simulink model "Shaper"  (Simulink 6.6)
settings: Solver=FixedStepDiscrete  StartTime=0.0  StopTime=1  FixedStep=0.001  RelTol=1e-3
PreLoadFcn:
  | load parameters
undefined symbols (not defined in the file or in its folder): f32_Traction_SlipShaperC, f32_Traction_SlipShaperDis, u32_Traction_SlipShaperOpt, u32_Traction_SlipShaperT

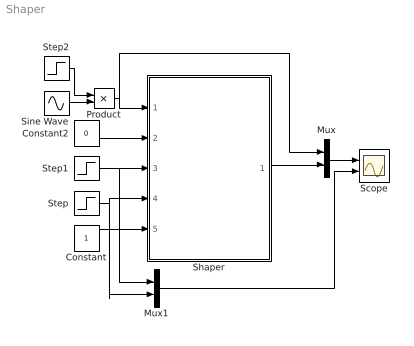
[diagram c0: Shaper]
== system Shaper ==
  Constant : Constant
  Constant2 : Constant  Value=0
  Mux : Mux  Inputs=2
  Mux1 : Mux  Inputs=2
  Product : Product
  Scope : Scope  NumInputPorts=2
  Shaper : Stateflow chart  TreatAsAtomicUnit=on
  Sine Wave : Sin  Amplitude=0.3  Bias=10  Frequency=2*pi  SampleTime=0
  Step : Step  Time=0.6  SampleTime=0
  Step1 : Step  Time=0.5  SampleTime=0
  Step2 : Step  Time=0.1  SampleTime=0
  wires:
  Constant/1 -> Shaper/5(EnableIn)
  Step/1 -> Shaper/4(Trigger), Mux1/2
  Constant2/1 -> Shaper/2(slip)
  Mux/1 -> Scope/1
  Shaper/1(out) -> Mux/2
  Step1/1 -> Shaper/3(CtrlActive), Mux1/1
  Mux1/1 -> Scope/2
  Product/1 -> Shaper/1(in), Mux/1
  Sine Wave/1 -> Product/2
  Step2/1 -> Product/1

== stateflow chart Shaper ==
  state Shaper [parallel]
    state PROCESS(N) [function]
      (junction 31) -> (junction 17)
      (junction 17) -> (junction 18) : [cnt < N] {j = MOD(j+u32_Traction_SlipShaperT[cnt],512); ... buf1[j] += f32_Traction_SlipShaperC[cnt+1]*(in-lev);}
      (junction 18) -> (junction 17) : {cnt++;}
      (junction 17) -> (junction 19)
      (default) -> (junction 31) : {cnt = 0;}
      (junction 30) -> (junction 19)
      (junction 20) -> (junction 30) : {cnt++;}
      (junction 30) -> (junction 20) : [cnt < N] {j = MOD(j+u32_Traction_SlipShaperT[cnt],512); ... buf2[j] += f32_Traction_SlipShaperC[cnt+1]*(in-lev);}
      (junction 31) -> (junction 30) : [bufSel]
    state c = MOD(a,b) [function]
      (default) -> (junction 33)
      (junction 33) -> (junction 34) : [a<b] {c=a;}
      (junction 33) -> (junction 34) : {c=a-b*floor(a/b);}
    state SHAPING /
      j = i;
      SETOUT();
      PROCESS(15);
      i = MOD(i+1,512);
      CtrlActiveOld = CtrlActive;
      EnableInOld = EnableIn;
    state SETOUT [function]
      (junction 21) -> (junction 22) : [bufSel] {tmp = f32_Traction_SlipShaperC[0] * (in-lev) + buf2[j] + lev; buf2[j] = 0;}
      (junction 21) -> (junction 22) : {tmp = f32_Traction_SlipShaperC[0] * (in-lev) + buf1[j] + lev; buf1[j] = 0;}
      (default) -> (junction 21)
      (junction 22) -> (junction 36) : {out = tmp;}
      (junction 22) -> (junction 36) : [u32_Traction_SlipShaperOpt && ... (tmp >= in - f32_Traction_SlipShaperDis)] {DisableShp = 1; out = in;}
    state b = SEL(a) [function]
      (default) -> (junction 28)
      (junction 28) -> (junction 29) : {b = 1; Pad1 = 1;}
      (junction 28) -> (junction 29) : [a] {b = 0; Pad2 = 1;}
    state DISABLED /
      out = in;
      CtrlActiveOld = CtrlActive;
      EnableInOld = EnableIn;
    (junction 15) -> (junction 37)
    (junction 16) -> (junction 15) : [(CtrlActive > CtrlActiveOld) ...  && bufAvailable] {ReadyToTrigg = 1;}
    (junction 15) -> SHAPING  : [ReadyToTrigg && Trigger] {lev = slip; bufSel = SEL(bufSel); ... bufAvailable--; ReadyToTrigg = 0; ... DisableShp = 0;}
    SHAPING  -> (junction 35)
    (junction 16) -> (junction 15) : [!CtrlActive] {ReadyToTrigg = 0;}
    (default) -> SHAPING 
    (junction 16) -> (junction 15)
    (junction 35) -> (junction 16)
    (junction 35) -> (junction 16) : [EnableIn && !EnableInOld] {bufAvailable = 0; ... Pad1 = 1; ... Pad2 = 1;}
    (junction 37) -> DISABLED  : [DisableShp]
    (junction 37) -> SHAPING 
    DISABLED  -> (junction 35)
  state ZeroPadding [parallel]
    state BUF2 /
      PADDING(2,32);
    state IDLE /
    state PADDING(SEL,N) [function]
      (junction 24) -> (junction 23) : {i = i + N;}
      (junction 27) -> (junction 24) : {cnt++;}
      (junction 25) -> (junction 26) : [cnt < N] {buf1[i + cnt] = 0;}
      (junction 24) -> (junction 27) : [cnt < N] {buf2[i + cnt] = 0;}
      (junction 25) -> (junction 23) : {i = i + N;}
      (junction 26) -> (junction 25) : {cnt++;}
      (junction 32) -> (junction 24)
      (junction 32) -> (junction 25) : [SEL==1]
      (default) -> (junction 32) : {cnt = 0;}
    state BUF1 /
      PADDING(1,32);
    BUF2  -> IDLE  : [i >= 512] {Pad2 = 0; bufAvailable++;}
    BUF2  -> BUF2 
    BUF1  -> BUF1 
    BUF1  -> IDLE  : [i >= 512] {Pad1 = 0; bufAvailable++;}
    (default) -> IDLE 
    IDLE  -> BUF1  : [Pad1] {i = 0;}
    IDLE  -> BUF2  : [Pad2 && !Pad1] {i = 0;}
